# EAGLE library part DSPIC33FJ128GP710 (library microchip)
dsPIC33FJ128GP710 edit this description Auto generated by make-symbol-device-package-bsdl.ulp Rev. 25 Source: dsPIC33FJ128GP710.bsd
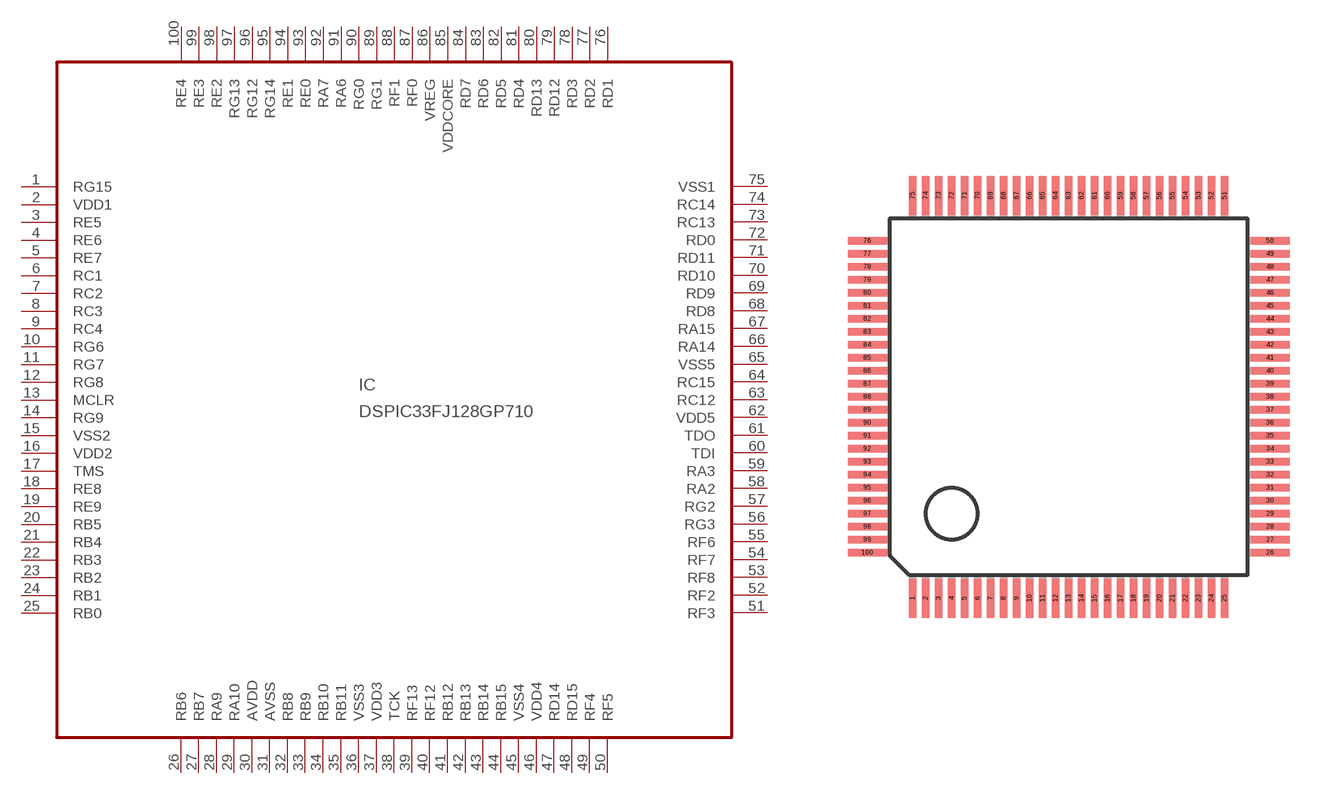
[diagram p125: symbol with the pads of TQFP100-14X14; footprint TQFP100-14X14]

Designator prefix IC

## DSPIC33FJ128GP710 (MPN: DSPIC33FJ128GP710-I/PF; OC_FARNELL: 1818690; OC_NEWARK: 74K4953)  [TQFP100-14X14]
1  RG15
2  VDD1  pwr
3  RE5
4  RE6
5  RE7
6  RC1
7  RC2
8  RC3
9  RC4
10  RG6
11  RG7
12  RG8
13  MCLR
14  RG9
15  VSS2  pwr
16  VDD2  pwr
17  TMS  in
18  RE8
19  RE9
20  RB5
21  RB4
22  RB3
23  RB2
24  RB1
25  RB0
26  RB6
27  RB7
28  RA9
29  RA10
30  AVDD  pwr
31  AVSS  pwr
32  RB8
33  RB9
34  RB10
35  RB11
36  VSS3  pwr
37  VDD3  pwr
38  TCK  in
39  RF13
40  RF12
41  RB12
42  RB13
43  RB14
44  RB15
45  VSS4  pwr
46  VDD4  pwr
47  RD14
48  RD15
49  RF4
50  RF5
51  RF3
52  RF2
53  RF8
54  RF7
55  RF6
56  RG3
57  RG2
58  RA2
59  RA3
60  TDI  in
61  TDO  out
62  VDD5  pwr
63  RC12
64  RC15
65  VSS5  pwr
66  RA14
67  RA15
68  RD8
69  RD9
70  RD10
71  RD11
72  RD0
73  RC13
74  RC14
75  VSS1  pwr
76  RD1
77  RD2
78  RD3
79  RD12
80  RD13
81  RD4
82  RD5
83  RD6
84  RD7
85  VDDCORE  pwr
86  VREG  pas
87  RF0
88  RF1
89  RG1
90  RG0
91  RA6
92  RA7
93  RE0
94  RE1
95  RG14
96  RG12
97  RG13
98  RE2
99  RE3
100  RE4

## Footprint TQFP100-14X14 (pad centres in mm)
Thin Quad Flat Pack 14x14 mm
smd 0.27 x 1.5: 1 -6,-7.75; 2 -5.5,-7.75; 3 -5,-7.75; 4 -4.5,-7.75; 5 -4,-7.75; 6 -3.5,-7.75; 7 -3,-7.75; 8 -2.5,-7.75; 9 -2,-7.75; 10 -1.5,-7.75; 11 -1,-7.75; 12 -0.5,-7.75; 13 0,-7.75; 14 0.5,-7.75; 15 1,-7.75; 16 1.5,-7.75; 17 2,-7.75; 18 2.5,-7.75; 19 3,-7.75; 20 3.5,-7.75; 21 4,-7.75; 22 4.5,-7.75; 23 5,-7.75; 24 5.5,-7.75; 25 6,-7.75; 51 6,7.75; 52 5.5,7.75; 53 5,7.75; 54 4.5,7.75; 55 4,7.75; 56 3.5,7.75; 57 3,7.75; 58 2.5,7.75; 59 2,7.75; 60 1.5,7.75; 61 1,7.75; 62 0.5,7.75; 63 0,7.75; 64 -0.5,7.75; 65 -1,7.75; 66 -1.5,7.75; 67 -2,7.75; 68 -2.5,7.75; 69 -3,7.75; 70 -3.5,7.75; 71 -4,7.75; 72 -4.5,7.75; 73 -5,7.75; 74 -5.5,7.75; 75 -6,7.75
smd 1.5 x 0.27: 26 7.75,-6; 27 7.75,-5.5; 28 7.75,-5; 29 7.75,-4.5; 30 7.75,-4; 31 7.75,-3.5; 32 7.75,-3; 33 7.75,-2.5; 34 7.75,-2; 35 7.75,-1.5; 36 7.75,-1; 37 7.75,-0.5; 38 7.75,0; 39 7.75,0.5; 40 7.75,1; 41 7.75,1.5; 42 7.75,2; 43 7.75,2.5; 44 7.75,3; 45 7.75,3.5; 46 7.75,4; 47 7.75,4.5; 48 7.75,5; 49 7.75,5.5; 50 7.75,6; 76 -7.75,6; 77 -7.75,5.5; 78 -7.75,5; 79 -7.75,4.5; 80 -7.75,4; 81 -7.75,3.5; 82 -7.75,3; 83 -7.75,2.5; 84 -7.75,2; 85 -7.75,1.5; 86 -7.75,1; 87 -7.75,0.5; 88 -7.75,0; 89 -7.75,-0.5; 90 -7.75,-1; 91 -7.75,-1.5; 92 -7.75,-2; 93 -7.75,-2.5; 94 -7.75,-3; 95 -7.75,-3.5; 96 -7.75,-4; 97 -7.75,-4.5; 98 -7.75,-5; 99 -7.75,-5.5; 100 -7.75,-6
